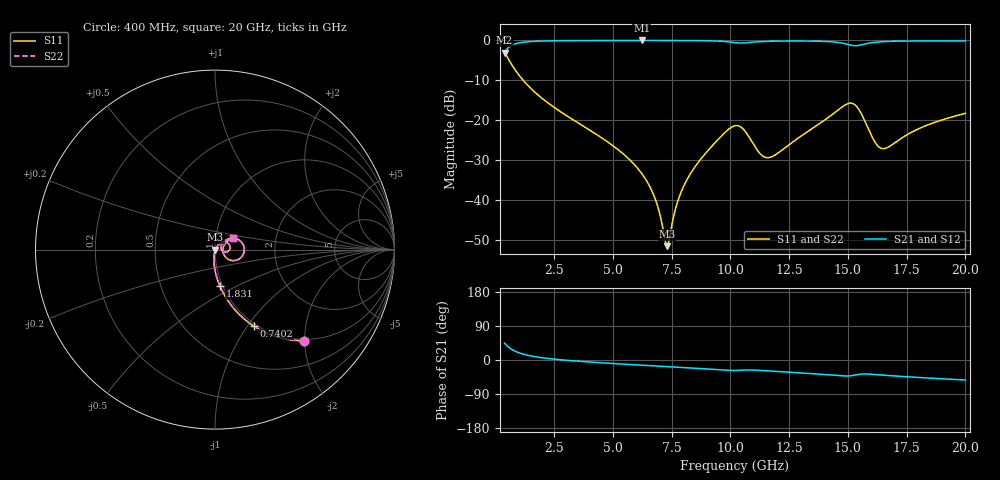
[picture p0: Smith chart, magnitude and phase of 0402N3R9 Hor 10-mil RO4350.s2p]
# GHz S MA R 50
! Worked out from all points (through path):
!   1960 points, 400 MHz to 20 GHz, reference 50 ohm
!   highest |S21| = -0.02 dB at 6.233 GHz (marker M1); lowest = -3.1 dB at 400 MHz (marker M2)
!   group delay of S21, straight-line fit = 9.25 ps
!   lowest |S11| = -51.6 dB at 7.314 GHz (marker M3), VSWR 1.01, Z = 50.2 - j0.0871 ohm
!   |S11| at or under -10 dB: 1.188 GHz to end of sweep
!   |S22| runs from -51.6 to -3.0 dB; largest |S21 - S12| = 0
!   S11 on the Smith chart (normalised r, x): 400 MHz: 0.97, -1.99; 740.2 MHz: 0.97, -1.07; 1.831 GHz: 0.97, -0.41; 20 GHz: 1.22, +0.16
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0.4  0.7102 -45.7  0.7035 44.3  0.7035 44.3  0.7102 -45.7
0.7401736  0.4765 -63.2  0.8784 26.7  0.8784 26.7  0.4765 -63.2
1.83073  0.2053 -82.2  0.9775 7.5  0.9775 7.5  0.2053 -82.2
3.671669  0.08666 -92.9  0.9947 -3.8  0.9947 -3.8  0.08666 -92.9
5.282491  0.0413 -98.0  0.9972 -10.3  0.9972 -10.3  0.0413 -98.0
6.232976  0.02133 -98.5  0.9976 -13.7  0.9976 -13.7  0.02133 -98.5
6.943338  0.007681 -88.7  0.9974 -16.1  0.9974 -16.1  0.007681 -88.7
7.313527  0.002619 -19.3  0.9971 -17.4  0.9971 -17.4  0.002619 -19.3
7.763757  0.009552 51.3  0.9964 -19.0  0.9964 -19.0  0.009552 51.3
8.223992  0.01942 56.5  0.9951 -20.7  0.9951 -20.7  0.01942 56.5
9.254518  0.04845 49.8  0.9855 -24.7  0.9855 -24.7  0.04845 49.8
10.205  0.08498 16.2  0.9365 -27.6  0.9365 -27.6  0.08498 16.2
10.53517  0.07786 -4.1  0.9272 -26.7  0.9272 -26.7  0.07786 -4.1
11.23553  0.03885 -8.4  0.9627 -27.3  0.9627 -27.3  0.03885 -8.4
11.5757  0.03372 9.7  0.9728 -28.5  0.9728 -28.5  0.03372 9.7
13.46667  0.07763 41.3  0.9795 -36.0  0.9795 -36.0  0.07763 41.3
15.17754  0.1625 -4.3  0.8644 -41.1  0.8644 -41.1  0.1625 -4.3
15.4977  0.1316 -26.9  0.8698 -37.6  0.8698 -37.6  0.1316 -26.9
16.24809  0.04832 -20.2  0.9534 -38.7  0.9534 -38.7  0.04832 -20.2
16.73834  0.04614 12.1  0.9709 -41.0  0.9709 -41.0  0.04614 12.1
18.12905  0.08068 34.0  0.9828 -46.5  0.9828 -46.5  0.08068 34.0
20  0.1214 32.7  0.9826 -52.9  0.9826 -52.9  0.1214 32.7
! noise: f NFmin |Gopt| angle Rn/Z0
0.4  0.001456  0.8136  2.21  0.001629
2.571  0.004721  0.659  6.883  0.002636
4.752  0.007224  0.6032  11.78  0.003327
6.933  0.0105  0.604  16.6  0.004803
9.104  0.02525  0.764  21.54  0.02098
11.29  0.05119  0.8501  26.66  0.06892
13.47  0.0388  0.7761  31.5  0.03286
15.64  0.1098  0.9028  36.5  0.2232
17.82  0.04117  0.7347  41.08  0.02727
20  0.03436  0.6634  45.35  0.01676
